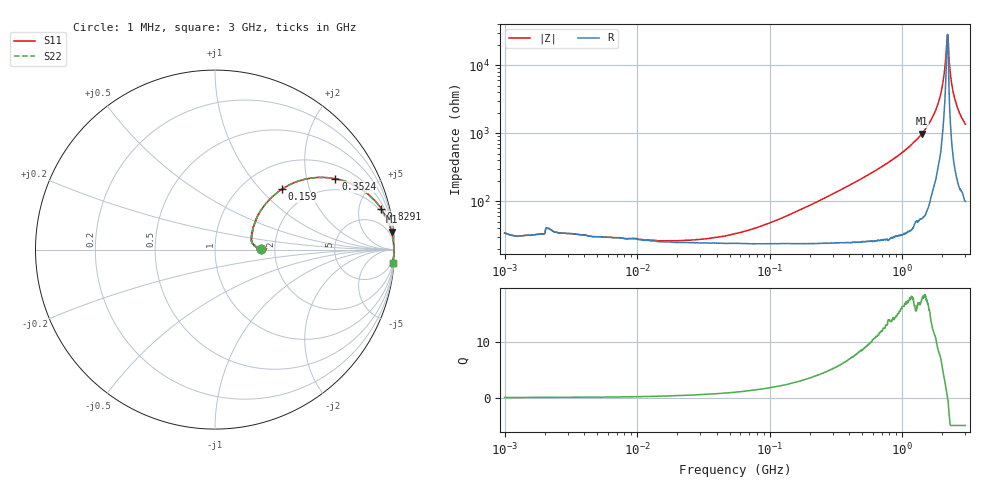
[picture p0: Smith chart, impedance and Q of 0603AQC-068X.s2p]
!s-Parameter Generated by FASTRON Sdn. Bhd.
!FASTRON P/N : 0603AQC-068X
!Keysight Technologies: E4991B_MY54100416_A.01.15
!Date: Thu Jun 25 13:55:00 2026
!Version  :Rev00  Thu Jun 25 13:55:00 2026
!Data & Calibration Information:
!Freq  S11  S21  S12  S22
!PortZ  Port1:50+j0  Port2:50+j0
!When reading reference impedance value at option line is always used.
! Remarks : This data is being provided solely for informational purposes.
# Hz S dB R 50
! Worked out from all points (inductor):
!   1601 points, 1 MHz to 3 GHz, reference 50 ohm
!   read as one part in series: L = 65.8 nH near 171.4 MHz
!   highest Q = 17.6 at 1.409 GHz (marker M1), where L = 112 nH
!   self-resonance near 2.2 GHz
!   S11 on the Smith chart (normalised r, x): 1 MHz: 1.68, +0.01; 159 MHz: 1.48, +1.33; 352.4 MHz: 1.49, +2.98; 829.1 MHz: 1.58, +7.95; 3 GHz: 3, -27
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1000000  -11.90 0.5  -2.55 -0.2  -2.55 -0.2  -11.90 0.5
1926146  -12.10 1.1  -2.47 -0.4  -2.47 -0.4  -12.10 1.1
2128890  -10.90 0.9  -2.92 -0.4  -2.92 -0.4  -10.90 0.9
3804036  -12.30 2.2  -2.42 -0.7  -2.42 -0.7  -12.30 2.2
1.447069e7  -13.60 11.0  -1.98 -2.9  -1.98 -2.9  -13.60 11.0
5.504702e7  -11.50 33.3  -2.02 -10.6  -2.02 -10.6  -11.50 33.3
1.590202e8  -5.99 42.1  -2.95 -28.2  -2.95 -28.2  -5.99 42.1
2.083556e8  -4.50 39.6  -3.60 -35.1  -3.60 -35.1  -4.50 39.6
3.523638e8  -2.18 30.5  -5.77 -50.1  -5.77 -50.1  -2.18 30.5
7.925923e8  -0.45 14.6  -12.00 -71.3  -12.00 -71.3  -0.45 14.6
8.291033e8  -0.41 13.8  -12.40 -72.0  -12.40 -72.0  -0.41 13.8
1.409185e9  -0.09 5.8  -20.00 -81.0  -20.00 -81.0  -0.09 5.8
1.67892e9  -0.06 3.4  -24.50 -82.2  -24.50 -82.2  -0.06 3.4
1.883708e9  -0.04 1.9  -29.30 -81.1  -29.30 -81.1  -0.04 1.9
2.01032e9  -0.03 1.1  -34.00 -78.4  -34.00 -78.4  -0.03 1.1
2.145442e9  -0.03 0.3  -43.70 -56.9  -43.70 -56.9  -0.03 0.3
2.188818e9  -0.03 0.1  -48.70 -18.3  -48.70 -18.3  -0.03 0.1
2.244273e9  -0.02 -0.3  -44.10 64.0  -44.10 64.0  -0.02 -0.3
2.359433e9  -0.02 -1.0  -34.80 80.9  -34.80 80.9  -0.02 -1.0
2.492946e9  -0.03 -1.8  -30.20 82.7  -30.20 82.7  -0.03 -1.8
2.714296e9  -0.05 -2.9  -25.90 82.6  -25.90 82.6  -0.05 -2.9
3e9  -0.07 -4.2  -22.70 81.6  -22.70 81.6  -0.07 -4.2
